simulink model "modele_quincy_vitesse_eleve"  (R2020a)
settings: Solver=VariableStepAuto  StartTime=0.0  StopTime=2  RelTol=1e-3
libraries: fl_lib x7, nesl_utility x3, ee_lib x1

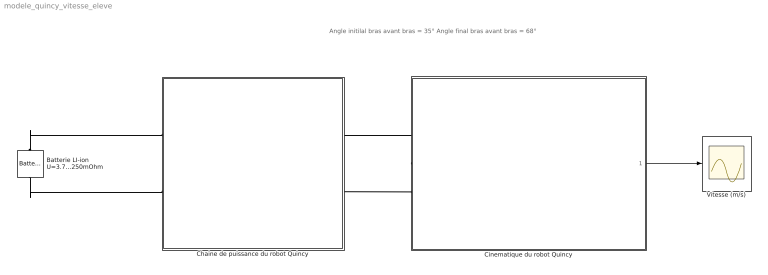
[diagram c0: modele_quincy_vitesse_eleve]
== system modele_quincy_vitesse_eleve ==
  note: Angle initilal bras avant bras = 35° Angle final bras avant bras = 68°
  Batterie LI-ion U=3.7V C=2.6A.h R=250mOhm : ee_lib/Sources/Battery  Vnom=3.7 V  R1=0.25 Ohm  prm_AH=1  AH=50 hr*A  V1=11.5 V  AH1=25 hr*A  prm_R2=1  R2=2000 Ohm  prm_dyn=1  Rp1=0.005 Ohm  tau1=30 s  Rp2=0.005 Ohm  tau2=30 s  Rp3=0.005 Ohm  tau3=30 s  Rp4=0.005 Ohm  tau4=30 s  Rp5=0.005 Ohm  tau5=30 s  prm_fade=1  N_fade=100  AH_fade=45 hr*A  R1_fade=2.02 Ohm  V1_fade=10.35 V  i_specify=off  i_priority=None  i=0 A  i_nominal_specify=off  i_nominal_unit=A  i_nominal_value=1  v_specify=off  v_priority=None  v=0 V  v_nominal_specify=off  v_nominal_unit=V  v_nominal_value=1  charge_specify=off  charge_priority=High  charge=50 hr*A  charge_nominal_specify=off  charge_nominal_unit=hr*A  charge_nominal_value=1  num_cycles_specify=off  num_cycles_priority=High  num_cycles=0  num_cycles_nominal_specify=off  num_cycles_nominal_unit=1  num_cycles_nominal_value=1  thermal_mass=30000 J/K  Tmeas=298.15 K  Vnom_T2=12 V  R1_T2=2.2 Ohm  V1_T2=11.4 V  R2_T2=2200 Ohm  Rp1_T2=0.005 Ohm  tau1_T2=30 s  Rp2_T2=0.005 Ohm  tau2_T2=30 s  Rp3_T2=0.005 Ohm  tau3_T2=30 s  Rp4_T2=0.005 Ohm  tau4_T2=30 s  Rp5_T2=0.005 Ohm  tau5_T2=30 s  Tmeas2=273.15 K  temperature_specify=off  temperature_priority=High  temperature=298.15 K  temperature_nominal_specify=off  temperature_nominal_unit=K  temperature_nominal_value=1
  Chaine de puissance du robot Quincy : Subsystem  mask{r=0}
      mask prompts: r "rapport de réduction (1/r)"
  Cinematique du robot Quincy : Subsystem  mask{e=0.11, L=0, alpha1=35, alpha2=68}
      mask prompts: e "Longueur bras (m)"; L "Longueur avant-bras (m)"; alpha1 "Angle initial (degrés)"; alpha2 "Angle final (degrés)"
  Vitesse (m/s) : Scope
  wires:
  Cinematique du robot Quincy/1(Out1) -> Vitesse (m/s)/1
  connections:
  Cinematique du robot Quincy/LConn1 -- Chaine de puissance du robot Quincy/RConn1
  Batterie LI-ion U=3.7V C=2.6A.h R=250mOhm/LConn1 -- Chaine de puissance du robot Quincy/LConn1
  Batterie LI-ion U=3.7V C=2.6A.h R=250mOhm/RConn1 -- Chaine de puissance du robot Quincy/LConn2
  Cinematique du robot Quincy/LConn2 -- Chaine de puissance du robot Quincy/RConn2

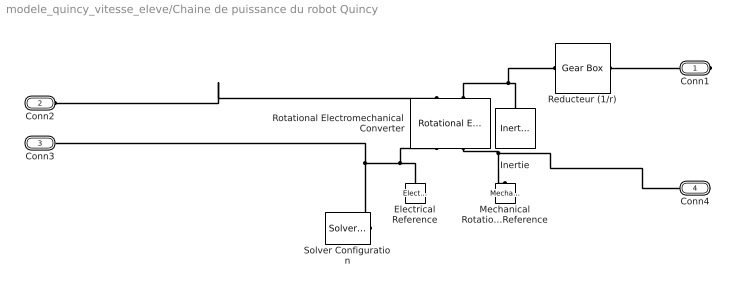
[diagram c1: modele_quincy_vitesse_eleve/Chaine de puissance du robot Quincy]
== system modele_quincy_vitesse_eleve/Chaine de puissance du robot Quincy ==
  Electrical Reference : fl_lib/Electrical/Electrical Elements/Electrical Reference
  Inertie : fl_lib/Mechanical/Rotational Elements/Inertia  inertia=0.013 kg*m^2  w_specify=off  w_priority=High  w=0 rad/s  w_nominal_specify=off  w_nominal_unit=rad/s  w_nominal_value=1  t_specify=off  t_priority=None  t=0 N*m  t_nominal_specify=off  t_nominal_unit=N*m  t_nominal_value=1
  Mechanical Rotational Reference : fl_lib/Mechanical/Rotational Elements/Mechanical Rotational Reference
  Reducteur (1/r) : fl_lib/Mechanical/Mechanisms/Gear Box  ratio=r  t_in_specify=off  t_in_priority=None  t_in=0 N*m  t_in_nominal_specify=off  t_in_nominal_unit=N*m  t_in_nominal_value=1  t_out_specify=off  t_out_priority=None  t_out=0 N*m  t_out_nominal_specify=off  t_out_nominal_unit=N*m  t_out_nominal_value=1
  Rotational Electromechanical Converter : fl_lib/Electrical/Electrical Elements/Rotational Electromechanical Converter  K=0.085*2.7 V/(rad/s)  i_specify=off  i_priority=None  i=0 A  i_nominal_specify=off  i_nominal_unit=A  i_nominal_value=1  v_specify=off  v_priority=None  v=0 V  v_nominal_specify=off  v_nominal_unit=V  v_nominal_value=1  t_specify=off  t_priority=None  t=0 N*m  t_nominal_specify=off  t_nominal_unit=N*m  t_nominal_value=1  w_specify=off  w_priority=None  w=0 rad/s  w_nominal_specify=off  w_nominal_unit=rad/s  w_nominal_value=1
  Solver Configuration : nesl_utility/Solver Configuration  PhysicalDomain=network_engine_domain  SubClassName=solver  LeftPortType=input  RightPortType=generic  Tones=[]  Harmonics=[]  SimulateNoise=off  Profile=off  UseLocalSampling=off  EnableSwitchedLinearOptims=on  FrequencyDomain=off  UseCCode=off  RelTol=0.001  AbsTol=1e-06  MinStep=1e-09  ToWorkspace=off  RevertToSquareIcSolve=off  NumHomotopyIterations=100  PhasorMode=off  PhasorModeNumHarmonics=1  DoDC=off  ResidualTolerance=1e-09  UseLocalSolver=off  LocalSolverChoice=NE_BACKWARD_EULER_ADVANCER  LocalSolverSampleTime=0.001  DoFixedCost=off  MaxNonlinIter=3  MaxModeIter=2  LinearAlgebra=Sparse  EquationFormulation=NE_TIME_EF  DelaysMemoryBudget=1024  AutomaticFiltering=on  FilteringTimeConstant=0.001  PartitionStorageMethod=AS_NEEDED  PartitionMemoryBudget=1024  PartitionMethod=FAST
  Conn1 : PMIOPort  Side=Right
  Conn2 : PMIOPort  Port=2  Side=Left
  Conn3 : PMIOPort  Port=3  Side=Left
  Conn4 : PMIOPort  Port=4  Side=Right
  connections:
  Conn2/RConn1 -- Rotational Electromechanical Converter/LConn1
  Solver Configuration/RConn1 -- Conn3/RConn1 -- Electrical Reference/LConn1 -- Rotational Electromechanical Converter/RConn1
  Rotational Electromechanical Converter/LConn2 -- Inertie/LConn1 -- Reducteur (1/r)/LConn1
  Rotational Electromechanical Converter/RConn2 -- Conn4/RConn1 -- Mechanical Rotational Reference/LConn1
  Conn1/RConn1 -- Reducteur (1/r)/RConn1

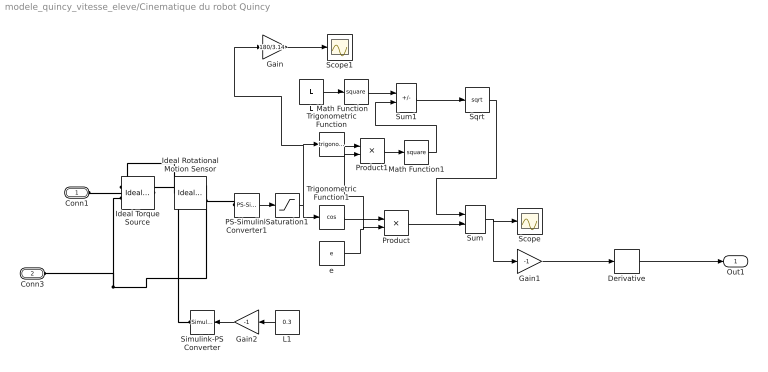
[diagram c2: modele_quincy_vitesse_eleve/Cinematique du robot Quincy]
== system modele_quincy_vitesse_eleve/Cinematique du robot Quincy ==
  Derivative : Derivative
  Gain : Gain  Gain=180/3.14
  Gain1 : Gain  Gain=-1
  Gain2 : Gain  Gain=-1
  Ideal Rotational Motion Sensor : fl_lib/Mechanical/Mechanical Sensors/Ideal Rotational Motion Sensor  wrap_angle=simscape.enum.onoff.off  offset=(35*3.14)/180 rad
  Ideal Torque Source : fl_lib/Mechanical/Mechanical Sources/Ideal Torque Source
  L : Constant  Value=L
  L1 : Constant  Value=0.3
  Math Function : Math  Operator=square  SignedPower=on
  Math Function1 : Math  Operator=square  SignedPower=on
  PS-Simulink Converter1 : nesl_utility/PS-Simulink Converter  PhysicalDomain=network_engine_domain  SubClassName=ps_output  LeftPortType=input  RightPortType=output  PseudoPeriodic=off  Frequencies=[]  Unit=rad  AffineConversion=off
  Product : Product
  Product1 : Product
  Saturation1 : Saturate  UpperLimit=(alpha2*3.14)/180  LowerLimit=(alpha1*3.14)/180
  Scope : Scope
  Scope1 : Scope
  Simulink-PS Converter : nesl_utility/Simulink-PS Converter  PhysicalDomain=network_engine_domain  SubClassName=ps_input  LeftPortType=input  RightPortType=output  PseudoPeriodic=off  Frequencies=[]  NoiseDistribution=none  NoiseParameters=[]  Unit=N*m  AffineConversion=off  FilteringAndDerivatives=provide  SimscapeFilterOrder=1  InputFilterTimeConstant=0.001  UdotUserProvided=0
  Sqrt : Sqrt
  Sum : Sum
  Sum1 : Sum  Inputs=+-
  Trigonometric Function : Trigonometry
  Trigonometric Function1 : Trigonometry  Operator=cos
  e : Constant  Value=e
  Conn1 : PMIOPort  Side=Left
  Conn3 : PMIOPort  Port=2  Side=Left
  Out1 : Outport  VectorParamsAs1DForOutWhenUnconnected=off
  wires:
  Product/1 -> Sum/2
  e/1 -> Product1/2, Product/2
  Product1/1 -> Math Function1/1
  Sum1/1 -> Sqrt/1
  Derivative/1 -> Out1/1
  Sum/1 -> Gain1/1, Scope/1
  Gain/1 -> Scope1/1
  Gain1/1 -> Derivative/1
  Trigonometric Function1/1 -> Product/1
  Trigonometric Function/1 -> Product1/1
  PS-Simulink Converter1/1 -> Saturation1/1
  L/1 -> Math Function/1
  Math Function/1 -> Sum1/1
  Sqrt/1 -> Sum/1
  Math Function1/1 -> Sum1/2
  Saturation1/1 -> Trigonometric Function1/1, Gain/1, Trigonometric Function/1
  L1/1 -> Gain2/1
  Gain2/1 -> Simulink-PS Converter/1
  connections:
  Ideal Torque Source/LConn1 -- Ideal Rotational Motion Sensor/LConn1 -- Conn1/RConn1
  Simulink-PS Converter/RConn1 -- Ideal Torque Source/RConn1
  Ideal Torque Source/RConn2 -- Conn3/RConn1 -- Ideal Rotational Motion Sensor/RConn1
  PS-Simulink Converter1/LConn1 -- Ideal Rotational Motion Sensor/RConn3
